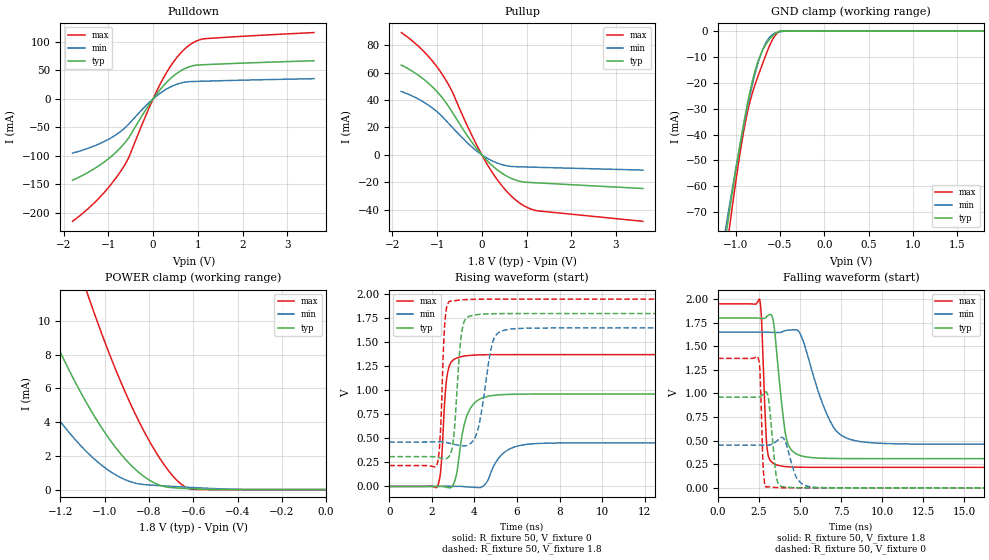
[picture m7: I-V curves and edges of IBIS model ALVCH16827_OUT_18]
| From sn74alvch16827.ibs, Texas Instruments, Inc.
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[Model]   ALVCH16827_OUT_18
Model_type  3-state
Enable   Active-Low
Vref =   0
Rref =   1000
Cref =   30p
Vmeas =   0.9
| variable   typ   min   max
C_comp   3.14pF   2.64pF   3.41pF
| C_pullup   4.25pF   3.42pF   4.91pF
| C_pulldown   8.98pF   4.90pF   12.96pF
| C_tri-state   3.14pF   2.64pF   3.41pF
[Temperature Range]   40   100   -40
| Ambient temperature   25   85   -40
[Voltage range]   1.8   1.65   1.95
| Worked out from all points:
|   slope of the pulldown table from 0 to 0.27 V, typ, clamps not added: 10.2 ohm
|   slope of the pullup table from 0 to 0.27 V, typ, clamps not added: 30.2 ohm
|   GND clamp passes 1 mA (typ) near -0.55 V on its own axis
|   POWER clamp passes 1 mA (typ) near -0.84 V on its own axis
|   rising waveform, R_fixture 50, V_fixture 0: 20-80 % time 501ps typ, 774ps min, 228ps max; typ from 0 V to 0.962 V
|   falling waveform, R_fixture 50, V_fixture 1.8: 20-80 % time 537ps typ, 1.41ns min, 234ps max; typ from 1.8 V to 0.31 V
|   rising waveform, R_fixture 50, V_fixture 1.8: 20-80 % time 282ps typ, 494ps min, 179ps max; typ from 0.31 V to 1.8 V
|   falling waveform, R_fixture 50, V_fixture 0: 20-80 % time 312ps typ, 520ps min, 149ps max; typ from 0.962 V to 0 V
[GND Clamp]
| ALVCH16827_OUT_18
|   Voltage   I(typ)   I(min)   I(max)
-1.8V     -255.4mA   -234.2mA   -289.8mA
-1.11V    -78.48mA   -75.46mA   -86.17mA
-1.09V    -73.85mA   -71.3mA    -80.88mA
-1.065V   -68.16mA   -66.17mA   -74.37mA
-915mV    -36.6mA    -37.4mA    -39.67mA
-865mV    -27.6mA    -28.89mA   -30.99mA
-805mV    -18.4mA    -19.73mA   -23.18mA
-750mV    -11.93mA   -12.67mA   -17.6mA
-685mV    -6.713mA   -6.416mA   -11.59mA
-570mV    -1.562mA   -1.092mA   -2.544mA
-485mV    -45.93uA   -285.5uA   -23.63uA
1.8V      1.168nA    69.01nA    28.27pA
[POWER Clamp]
| ALVCH16827_OUT_18
|   Voltage   I(typ)   I(min)   I(max)
-1.8V     29.67mA    18.6mA     47.93mA
-1.545V   19.46mA    11.49mA    33.45mA
-1.31V    11.36mA    6.08mA     21.55mA
-1.19V    7.854mA    3.858mA    16.15mA
-1.07V    4.862mA    2.091mA    11.3mA
-925mV    2.076mA    692.7uA    6.307mA
-850mV    1.061mA    349.8uA    4.157mA
-770mV    359.1uA    250.1uA    2.24mA
-695mV    116.6uA    190uA      848.9uA
-635mV    67.93uA    145.8uA    152.5uA
-585mV    37.09uA    111uA      9.499uA
-16.28fV  1.168nA    59.88nA    33.87pA
[Pulldown]
| ALVCH16827_OUT_18
|   Voltage   I(typ)   I(min)   I(max)
-1.8V     -142.5mA   -94.94mA   -214.6mA
-1.19V    -116mA     -78.24mA   -172.4mA
-925mV    -100.2mA   -67.56mA   -148.5mA
-690mV    -82.3mA    -54.81mA   -122.9mA
-535mV    -66.97mA   -43.32mA   -101mA
-105mV    -12.13mA   -7.634mA   -18.73mA
200mV     20.41mA    12.38mA    32.16mA
490mV     42.45mA    24.65mA    68.46mA
785mV     55.72mA    30.25mA    92.88mA
970mV     59.35mA    30.84mA    101.8mA
1.155V    60.2mA     31.26mA    105.7mA
3.6V      67.09mA    35.62mA    116.5mA
[Pullup]
| ALVCH16827_OUT_18
|   Voltage   I(typ)   I(min)   I(max)
-1.8V     65.54mA    46.25mA    89.25mA
-1.32V    55.67mA    38.89mA    76.19mA
-1.11V    49.72mA    34.29mA    68.65mA
-920mV    43.05mA    29.01mA    60.43mA
-685mV    32.34mA    20.89mA    47.55mA
-250mV    10.47mA    6.526mA    16.03mA
115mV     -4.131mA   -2.38mA    -6.642mA
450mV     -13.44mA   -7.131mA   -22.64mA
790mV     -18.81mA   -8.709mA   -33.84mA
1.02V     -20.1mA    -8.918mA   -38.54mA
1.25V     -20.5mA    -9.124mA   -40.92mA
3.6V      -24.58mA   -11.14mA   -48.53mA
[Ramp]
| ALVCH16827_OUT_18
| variable   typ   min   max
dV/dt_r   0.59/5.13E-10   0.28/7.76E-10   0.83/2.48E-10
dV/dt_f   0.92/5.50E-10   0.73/1.43E-09   1.07/2.48E-10
R_load = 50
[Rising Waveform]
| ALVCH16827_OUT_18
R_fixture =   50
C_fixture =   0
L_fixture =   0
V_fixture =   0
V_fixture_min = 0
V_fixture_max = 0
|   Time   V(typ)   V(min)   V(max)
0s        271.6pV    1.336nV    199.1pV
2.255ns   1.953mV    -256.9uV   -2.743mV
2.415ns   1.548mV    162.6uV    161.3mV
2.625ns   -5.104mV   1.333mV    952.9mV
2.775ns   -12.49mV   1.421mV    1.219V
3.135ns   101.7mV    902.1uV    1.333V
3.62ns    718.3mV    -4.19mV    1.36V
4.45ns    926.6mV    9.405mV    1.371V
7.045ns   961.5mV    447.8mV    1.372V
50ns      961.7mV    453.8mV    1.372V
[Falling Waveform]
| ALVCH16827_OUT_18
R_fixture =   50
C_fixture =   0
L_fixture =   0
V_fixture =   1.8
V_fixture_min = 1.65
V_fixture_max = 1.95
|   Time   V(typ)   V(min)   V(max)
0s        1.8V       1.65V      1.95V
2.535ns   1.798V     1.65V      1.996V
3ns       1.819V     1.65V      405mV
3.365ns   1.769V     1.647V     261.9mV
3.795ns   1.03V      1.647V     233.1mV
4.155ns   529.2mV    1.668V     224.8mV
4.585ns   381.7mV    1.674V     220.5mV
7.01ns    311.8mV    650mV      217.2mV
8.695ns   310mV      489.6mV    217.2mV
50ns      309.8mV    462.1mV    217.2mV
[Rising Waveform]
| ALVCH16827_OUT_18
R_fixture =   50
C_fixture =   0
L_fixture =   0
V_fixture =   1.8
V_fixture_min = 1.65
V_fixture_max = 1.95
|   Time   V(typ)   V(min)   V(max)
0s        309.8mV    462.1mV    217.2mV
2.23ns    304.7mV    464mV      219mV
2.4ns     295.9mV    465.7mV    546.6mV
2.625ns   287.6mV    460.7mV    1.74V
2.91ns    359.3mV    444.4mV    1.931V
3.425ns   1.634V     422.6mV    1.943V
4.095ns   1.788V     542.9mV    1.949V
4.875ns   1.798V     1.513V     1.95V
5.745ns   1.8V       1.64V      1.95V
50ns      1.8V       1.65V      1.95V
[Falling Waveform]
| ALVCH16827_OUT_18
R_fixture =   50
C_fixture =   0
L_fixture =   0
V_fixture =   0
V_fixture_min = 0
V_fixture_max = 0
|   Time   V(typ)   V(min)   V(max)
0s        961.7mV    453.8mV    1.372V
2.44ns    960.7mV    452.6mV    1.378V
2.555ns   965.2mV    452.3mV    1.23V
2.77ns    997.3mV    451.5mV    160.3mV
2.97ns    1.011V     450.9mV    7.463mV
3.575ns   97.04mV    496.1mV    3.408mV
4.125ns   8.417mV    478.1mV    986.9uV
4.825ns   1.813mV    94.28mV    234.5uV
5.93ns    277.6uV    5.853mV    28.26uV
50ns      695.2pV    681.7pV    1.699nV
